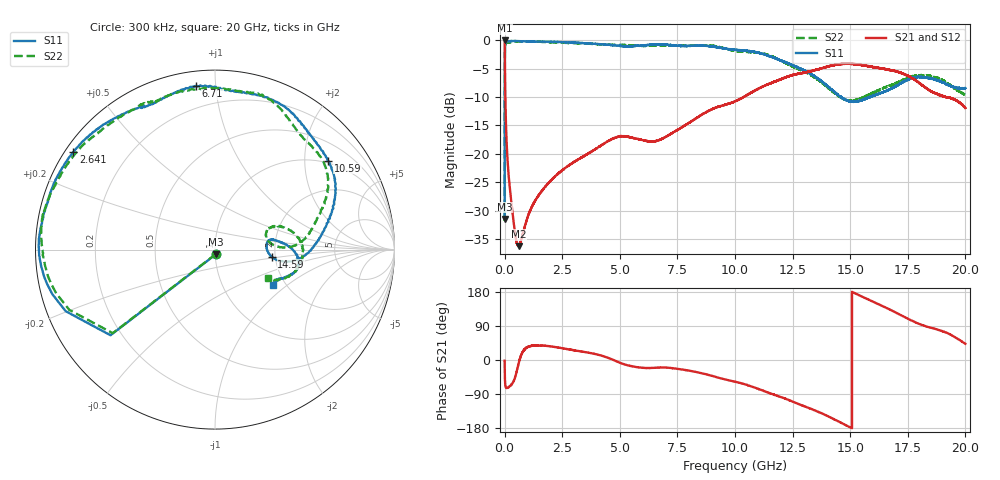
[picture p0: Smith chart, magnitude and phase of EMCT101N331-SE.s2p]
!EMCT101N331
!Johanson Technology Inc.
!www.johansontechnology.com
!Test Board Conditions:
!Substrate Type  RO4350B
!Substrate Thickness  10 mil
!Substrate Dk  3.66
!TL Type: GCPW
!TL Trace Width  22 mil
!TL Gap  14 mil
!PART MODE SINGLE ENDED (AKA BYPASS)
!DUT TOPOLOGY	SERIES-SHUNT
# MHz S  dB  R 50
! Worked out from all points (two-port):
!   20001 points, 300 kHz to 20 GHz, reference 50 ohm
!   highest |S21| = -0.06 dB at 300 kHz (marker M1); lowest = -36.2 dB at 614.3 MHz (marker M2)
!   |S21| within 3 dB of the highest: start of sweep to 10.81 MHz
!   lowest |S11| = -31.4 dB at 300 kHz (marker M3), VSWR 1.06, Z = 50.4 - j2.66 ohm
!   |S11| at or under -10 dB: start of sweep to 3.754 MHz; 14.6 GHz to 15.86 GHz (1.254 GHz wide, 8.23 % of centre); 15.86106 GHz to 15.86106 GHz (0 Hz wide, 0 % of centre)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
!   |S22| runs from -31.8 to -0.2 dB; largest |S21 - S12| = 0.015
!   S11 on the Smith chart (normalised r, x): 300 kHz: 1.01, -0.05; 2.641 GHz: 0.02, +0.31; 6.71 GHz: 0.08, +0.89; 10.59 GHz: 0.93, +2.60; 14.59 GHz: 1.91, -0.17; 20 GHz: 1.73, -0.79
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0.3  -31.43 -80.0  -0.06 -1.6  -0.03 -1.5  -31.79 -81.8
107.298  -0.23 -175.2  -19.60 -73.7  -19.55 -73.9  -0.42 -174.9
187.297  -0.18 -178.6  -24.37 -71.1  -24.34 -71.1  -0.36 -178.1
342.295  -0.15 178.3  -30.25 -61.3  -30.26 -61.5  -0.31 178.3
614.291  -0.17 174.2  -36.21 -8.1  -36.20 -8.1  -0.23 174.0
1385.279  -0.27 163.7  -27.82 38.4  -27.80 38.8  -0.26 163.4
2641.26  -0.36 145.5  -22.43 29.5  -22.40 29.3  -0.47 147.2
3334.25  -0.51 136.4  -20.63 22.4  -20.62 22.4  -0.57 140.7
4959.226  -0.96 116.7  -16.95 -6.1  -16.98 -6.1  -0.89 120.4
6667.2  -0.76 97.0  -17.62 -20.0  -17.59 -20.4  -0.93 105.5
6710.199  -0.75 96.6  -17.55 -19.9  -17.51 -20.3  -0.91 104.9
8773.168  -1.01 66.4  -12.62 -38.1  -12.65 -38.3  -0.95 74.0
10000.15  -1.70 47.7  -10.75 -57.4  -10.60 -57.6  -1.87 55.2
10589.14  -1.91 38.1  -9.51 -67.1  -9.51 -68.1  -2.08 46.0
11615.13  -2.98 20.9  -7.48 -89.9  -7.46 -89.0  -2.89 28.6
13334.1  -6.06 -4.1  -5.42 -129.8  -5.44 -129.9  -6.24 5.4
14585.08  -9.95 -7.0  -4.21 -164.9  -4.21 -164.7  -10.08 6.1
15458.07  -10.63 8.0  -4.34 168.9  -4.28 168.8  -10.22 19.9
16667.05  -8.75 6.7  -5.21 134.7  -5.31 134.9  -8.07 18.7
17431.04  -7.07 -1.3  -6.15 111.1  -6.12 112.3  -6.77 10.2
18277.03  -6.62 -13.9  -8.35 89.0  -8.28 88.7  -6.25 -5.8
20000  -8.43 -31.2  -11.92 42.9  -12.05 44.0  -9.59 -28.1
